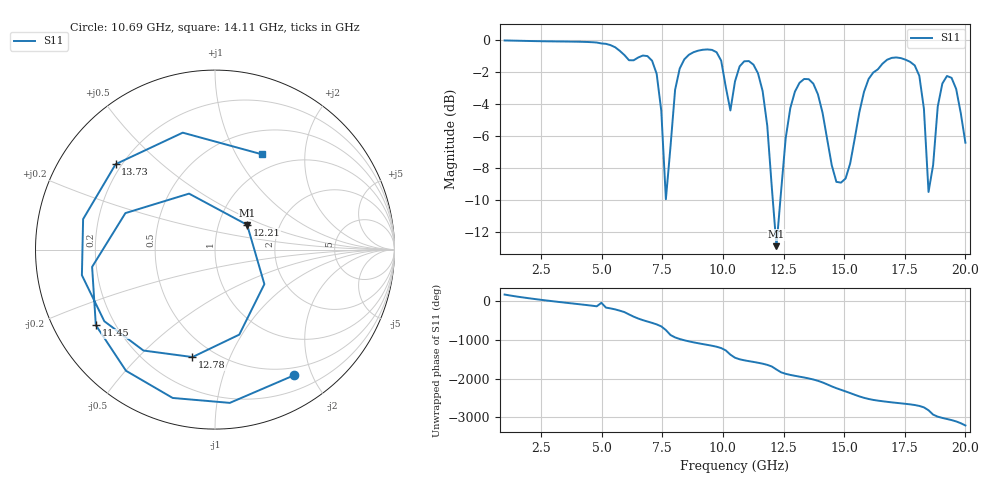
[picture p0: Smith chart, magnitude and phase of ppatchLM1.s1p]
# GHZ S RI R 50
!Output file by EM3DS_5.0
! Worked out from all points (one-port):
!   101 points, 1 GHz to 20 GHz, reference 50 ohm
!   lowest |S11| = -12.9 dB at 12.21 GHz (marker M1), VSWR 1.58, Z = 68.5 + j19.9 ohm
!   |S11| at or under -10 dB: 12.06 GHz to 12.37 GHz (313.6 MHz wide, 2.57 % of centre)
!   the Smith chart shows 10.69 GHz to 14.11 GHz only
!   S11 on the Smith chart (normalised r, x): 10.69 GHz: 0.39, -1.74; 11.45 GHz: 0.13, -0.29; 12.21 GHz: 1.37, +0.40; 12.78 GHz: 0.39, -0.74; 13.73 GHz: 0.18, +0.36; 14.11 GHz: 0.79, +1.29
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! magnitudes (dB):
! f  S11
! 1 GHz  0.0
! 3.47 GHz  -0.1
! 5.75 GHz  -0.7
! 7.27 GHz  -2.1
! 7.46 GHz  -4.4
! 7.65 GHz  -10.0
! 8.22 GHz  -1.8
! 9.74 GHz  -0.8
! 10.31 GHz  -4.4
! 10.5 GHz  -2.6
! 10.69 GHz  -1.6
! 11.45 GHz  -2.1
! 11.83 GHz  -5.4
! 12.21 GHz  -12.9
! 12.78 GHz  -4.3
! 12.97 GHz  -3.2
! 13.73 GHz  -2.7
! 14.11 GHz  -4.6
! 14.68 GHz  -8.9
! 15.44 GHz  -6.1
! 16.2 GHz  -2.0
! 17.72 GHz  -1.4
! 18.1 GHz  -2.2
! 18.29 GHz  -4.3
! 18.48 GHz  -9.5
! 18.86 GHz  -4.2
! 19.24 GHz  -2.3
! 20 GHz  -6.4
